| IBIS file stm32l4p5_wlcsp100_p.ibs
[IBIS ver]   4.2
[File name]  stm32l4p5_wlcsp100_p.ibs
[File Rev]   1.0
[Date]   04-10-2019
[Source]   Data Created at STMicroelectronics
[Notes]   File originated from ELDO simulations.
[Disclaimer] This information is for modeling purpose only and is
   not guaranted.
   The information is subject to change without notice.
[Copyright]  Copyright 2019 STMicroelectronics Inc.
|   Component stm32l4p5_wlcsp100_p
[Component] stm32l4p5_wlcsp100_p
[Manufacturer] STMicroelectronics
[Package]
| variable   typ   min   max
R_pkg  0  NA  NA
L_pkg  0  NA  NA
C_pkg  0  NA  NA
[Pin]   signal_name   model_name R_pin L_pin C_pin
A1 VDDUSB POWER
A10 VDD POWER
A2 PA15 io8prog2m25m50m120m_sudq_ft
A3 PD1 io8prog2m25m50m120m_sudq_ft
A4 VDD POWER
A5 PG10 io8prog2m25m50m120m_sudq_ft
A6 VDDIO2 POWER
A7 PB6 io8prog2m25m50m120m_sudq_i2c_ft
A8 PB9 io8prog2m25m50m120m_sudq_i2c_ft
A9 VDD12 POWER
B1 VSS GND
B10 PE3 io8prog2m25m50m120m_sudq_ft
B2 PA14 io8prog2m25m50m120m_sudq_ft
B3 PD0 io8prog2m25m50m120m_sudq_ft
B4 PD5 io8prog2m25m50m120m_sudq_ft
B5 PD6 io8prog2m25m50m120m_sudq_ft
B6 PG12 io8prog2m25m50m120m_sudq_ft
B7 PB7 io8prog2m25m50m120m_sudq_i2c_ft
B8 PB8 io8prog2m25m50m120m_sudq_i2c_ft
B9 VSS GND
C1 PA12 io8usblsfs_otg2
C10 VBAT POWER
C2 PA13 io8prog2m25m50m120m_sudq_ft
C3 PC10 io8prog2m25m50m120m_sudq_ft
C4 PC12 io8prog2m25m50m120m_sudq_ft
C5 PD4 io8prog2m25m50m120m_sudq_ft
C6 PD7 io8prog2m25m50m120m_sudq_ft
C7 PB5 io8prog2m25m50m120m_sudq_ft
C8 PE2 io8prog2m25m50m120m_sudq_ft
C9 PC13 io8prog2m25m50m120m_sudq_ft
D1 PA11 io8usblsfs_otg2
D10 PC14-OSC32_IN io8prog2m25m50m120m_sudq_ft
D2 PA10 io8usb_id_otg20_lcd4_ft_ms
D3 PA9 POWER
D4 PC11 io8prog2m25m50m120m_sudq_ft
D5 PD2 io8prog2m25m50m120m_sudq_ft
D6 PG9 io8prog2m25m50m120m_sudq_ft
D7 PH3-BOOT0 io8prog2m25m50m120m_sudq_ft
D8 PE6 io8prog2m25m50m120m_sudq_ft
D9 PC15-OSC32_OUT io8prog2m25m50m120m_sudq_ft
E1 PC8 io8prog2m25m50m120m_sudq_ft
E10 VSS GND
E2 PC9 io8prog2m25m50m120m_sudq_ft
E3 PA8 io8prog2m25m50m120m_sudq_ft
E4 PC7 io8prog2m25m50m120m_sudq_ft
E5 PG11 io8prog2m25m50m120m_sudq_ft
E6 PB4 io8prog2m25m50m120m_sudq_ft
E7 PE4 io8prog2m25m50m120m_sudq_ft
E8 PE5 io8prog2m25m50m120m_sudq_ft
E9 VDD POWER
F1 VDD POWER
F10 PH0-OSC_IN io8prog2m25m50m120m_sudq_ft
F2 PD15 io8prog2m25m50m120m_sudq_ft
F3 PD14 io8prog2m25m50m120m_sudq_ft
F4 PC6 io8prog2m25m50m120m_sudq_ft
F5 PB3 io8prog2m25m50m120m_sudq_ft
F6 PC3 io8prog2m25m50m120m_sudq_ft
F7 PC1 io8prog2m25m50m120m_sudq_i2c_ft
F8 NRST ioreset_ft_v33
F9 PH1-OSC_OUT io8prog2m25m50m120m_sudq_ft
G1 PD10 io8prog2m25m50m120m_sudq_ft
G10 PC0 io8prog2m25m50m120m_sudq_i2c_ft
G2 PD9 io8prog2m25m50m120m_sudq_ft
G3 PD8 io8prog2m25m50m120m_sudq_ft
G4 PE14 io8prog2m25m50m120m_sudq_ft
G5 PE13 io8prog2m25m50m120m_sudq_ft
G6 PA7 io8prog2m25m50m120m_sudq_ft
G7 PA1 io8prog2m25m50m120m_sudq_ft
G8 PA0 io8prog2m25m50m120m_sudq_ft
G9 PC2 io8prog2m25m50m120m_sudq_ft
H1 PB14 io8prog2m25m50m120m_sudq_i2c_ft
H10 VREF+ POWER
H2 PB13 io8prog2m25m50m120m_sudq_i2c_ft
H3 PB15 io8prog2m25m50m120m_sudq_ft
H4 PE15 io8prog2m25m50m120m_sudq_ft
H5 PE10 io8prog2m25m50m120m_sudq_ft
H6 PB0 io8prog2m25m50m120m_sudq_ft
H7 PA4 io8prog2m25m50m120m_sudq_ft
H8 PA2 io8prog2m25m50m120m_sudq_ft
H9 VSSA GND
J1 PB12 io8w_swp_lcd4_ft
J10 VDDA POWER
J2 VDD POWER
J3 PB11 io8prog2m25m50m120m_sudq_i2c_ft
J4 PE12 io8prog2m25m50m120m_sudq_ft
J5 PE9 io8prog2m25m50m120m_sudq_ft
J6 PB2 io8prog2m25m50m120m_sudq_ft
J7 PA5 io8prog2m25m50m120m_sudq_ft
J8 VDD POWER
J9 PA3 io8prog2m25m50m120m_sudq_ft
K1 VDD12 GND
K10 VSS GND
K2 VSS GND
K3 PB10 io8prog2m25m50m120m_sudq_i2c_ft
K4 PE11 io8prog2m25m50m120m_sudq_ft
K5 PE8 io8prog2m25m50m120m_sudq_ft
K6 PE7 io8prog2m25m50m120m_sudq_ft
K7 PB1 io8prog2m25m50m120m_sudq_ft
K8 PC4 io8prog2m25m50m120m_sudq_ft
K9 PA6 io8prog2m25m50m120m_sudq_ft
[Model Selector] io8prog2m25m50m120m_sudq_ft
iols8p_sudq_ft_pd_lv  "IO low speed, PD=40kOhm - 1P8V"
iols8p_sudq_ft_pu_lv  "IO low speed, PU=40kOhm - 1P8V"
iols8p_sudq_ft_lv  "IO low speed - 1P8V"
iols8p_sudq_ft_pd  "IO low speed, PD=40kOhm - 3P3V"
iols8p_sudq_ft_pu  "IO low speed, PU=40kOhm - 3P3V"
iols8p_sudq_ft  "IO low speed - 3P3V"
iofs8p_sudq_ft_pd_lv  "IO full speed, PD=40kOhm - 1P8V"
iofs8p_sudq_ft_pu_lv  "IO full speed, PU=40kOhm - 1P8V"
iofs8p_sudq_ft_lv  "IO full speed - 1P8V"
iofs8p_sudq_ft_pd  "IO full speed, PD=40kOhm - 3P3V"
iofs8p_sudq_ft_pu  "IO full speed, PU=40kOhm - 3P3V"
iofs8p_sudq_ft  "IO full speed - 3P3V"
ioms8p_sudq_ft_pd_lv  "IO medium speed, PD=40kOhm - 1P8V"
ioms8p_sudq_ft_pu_lv  "IO medium speed, PU=40kOhm - 1P8V"
ioms8p_sudq_ft_lv  "IO medium speed - 1P8V"
ioms8p_sudq_ft_pd  "IO medium speed, PD=40kOhm - 3P3V"
ioms8p_sudq_ft_pu  "IO medium speed, PU=40kOhm - 3P3V"
ioms8p_sudq_ft  "IO medium speed - 3P3V"
iohs8p_sudq_ft_pd_lv  "IO high speed, PD=40kOhm - 1P8V"
iohs8p_sudq_ft_pu_lv  "IO high speed, PU=40kOhm - 1P8V"
iohs8p_sudq_ft_lv  "IO high speed - 1P8V"
iohs8p_sudq_ft_pd  "IO high speed, PD=40kOhm - 3P3V"
iohs8p_sudq_ft_pu  "IO high speed, PU=40kOhm - 3P3V"
iohs8p_sudq_ft  "IO high speed - 3P3V"
[Model Selector] io8prog2m25m50m120m_sudq_i2c_ft
io8prog_1v8_i2c_pd  "5V Tol GPIO 1.8V range i2c functionality with pull down"
io8prog_1v8_i2c_pu  "5V Tol GPIO 1.8V range i2c functionality with pull up"
io8prog_1v8_i2c  "5V Tol GPIO 1.8V range i2c functionality"
io8prog_3v3_i2c_pd  "5V Tol GPIO 3.3V range i2c functionality with pull down"
io8prog_3v3_i2c_pu  "5V Tol GPIO 3.3V range i2c functionality with pull up"
io8prog_3v3_i2c  "5V Tol GPIO 3.3V range i2c functionality"
iols8p_sudq_ft_pd_lv  "IO low speed, PD=40kOhm - 1P8V"
iols8p_sudq_ft_pu_lv  "IO low speed, PU=40kOhm - 1P8V"
iols8p_sudq_ft_lv  "IO low speed - 1P8V"
iols8p_sudq_ft_pd  "IO low speed, PD=40kOhm - 3P3V"
iols8p_sudq_ft_pu  "IO low speed, PU=40kOhm - 3P3V"
iols8p_sudq_ft  "IO low speed - 3P3V"
iofs8p_sudq_ft_pd_lv  "IO full speed, PD=40kOhm - 1P8V"
iofs8p_sudq_ft_pu_lv  "IO full speed, PU=40kOhm - 1P8V"
iofs8p_sudq_ft_lv  "IO full speed - 1P8V"
iofs8p_sudq_ft_pd  "IO full speed, PD=40kOhm - 3P3V"
iofs8p_sudq_ft_pu  "IO full speed, PU=40kOhm - 3P3V"
iofs8p_sudq_ft  "IO full speed - 3P3V"
ioms8p_sudq_ft_pd_lv  "IO medium speed, PD=40kOhm - 1P8V"
ioms8p_sudq_ft_pu_lv  "IO medium speed, PU=40kOhm - 1P8V"
ioms8p_sudq_ft_lv  "IO medium speed - 1P8V"
ioms8p_sudq_ft_pd  "IO medium speed, PD=40kOhm - 3P3V"
ioms8p_sudq_ft_pu  "IO medium speed, PU=40kOhm - 3P3V"
ioms8p_sudq_ft  "IO medium speed - 3P3V"
iohs8p_sudq_ft_pd_lv  "IO high speed, PD=40kOhm - 1P8V"
iohs8p_sudq_ft_pu_lv  "IO high speed, PU=40kOhm - 1P8V"
iohs8p_sudq_ft_lv  "IO high speed - 1P8V"
iohs8p_sudq_ft_pd  "IO high speed, PD=40kOhm - 3P3V"
iohs8p_sudq_ft_pu  "IO high speed, PU=40kOhm - 3P3V"
iohs8p_sudq_ft  "IO high speed - 3P3V"
[Model Selector] io8w_swp_lcd4_ft
io8w_swp_classc  "Class C swp functionality"
io8w_swp_classb  "Class B swp functionality"
io8lsw_1v8_pd  "GPIO 1.8V range with pd io low speed"
io8lsw_1v8_pu  "GPIO 1.8V range with pu io low speed"
io8lsw_1v8  "GPIO 1.8V range io low speed"
io8lsw_3v3_pd  "GPIO 3.3V range with pd io low speed"
io8lsw_3v3_pu  "GPIO 3.3V range with pu io low speed"
io8lsw_3v3  "GPIO 3.3V range io low speed"
io8fsw_1v8_pd  "GPIO 1.8V range with pd io full speed"
io8fsw_1v8_pu  "GPIO 1.8V range with pu io full speed"
io8fsw_1v8  "GPIO 1.8V range io full speed"
io8fsw_3v3_pd  "GPIO 3.3V range with pd io full speed"
io8fsw_3v3_pu  "GPIO 3.3V range with pu io full speed"
io8fsw_3v3  "GPIO 3.3V range io full speed"
io8msw_1v8_pd  "GPIO 1.8V range with pd io medium speed"
io8msw_1v8_pu  "GPIO 1.8V range with pu io medium speed"
io8msw_1v8  "GPIO 1.8V range io medium speed"
io8msw_3v3_pd  "GPIO 3.3V range with pd io medium speed"
io8msw_3v3_pu  "GPIO 3.3V range with pu io medium speed"
io8msw_3v3  "GPIO 3.3V range io medium speed"
io8hsw_1v8_pd  "GPIO 1.8V range with pd io high speed"
io8hsw_1v8_pu  "GPIO 1.8V range with pu io high speed"
io8hsw_1v8  "GPIO 1.8V range io high speed"
io8hsw_3v3_pd  "GPIO 3.3V range with pd io high speed"
io8hsw_3v3_pu  "GPIO 3.3V range with pu io high speed"
io8hsw_3v3  "GPIO 3.3V range io high speed"
[Model Selector] io8usblsfs_otg2
usb_ls_pd  "USB Low Speed mode - Pull Down"
usb_ls_pu2  "USB Low Speed mode - Pull up 2"
usb_ls_pu  "USB Low Speed mode - Pull up"
usb_fs  "USB Low Speed mode"
usb_fs_pd  "USB Full Speed mode - Pull Down"
usb_fs_pu2  "USB Full Speed mode - Pull up 2"
usb_fs_pu  "USB Full Speed mode - Pull up"
[Model Selector] io8usb_id_otg20_lcd4_ft_ms
io8usbid_1v8_id_pu  "ID 1V8 range with pull up"
io8usbid_3v3_id_pu  "ID 3V3 range with pull up"
io8usbid_1v8_id  "ID 1V8 range"
io8usbid_3v3_id  "ID 3V3 range"
io8lsusbid_1v8_pd  "GPIO 1.8V range with pd io low speed"
io8lsusbid_1v8_pu  "GPIO 1.8V range with pu io low speed"
io8lsusbid_1v8  "GPIO 1.8V range io low speed"
io8lsusbid_3v3_pd  "GPIO 3.3V range with pd io low speed"
io8lsusbid_3v3_pu  "GPIO 3.3V range with pu io low speed"
io8lsusbid_3v3  "GPIO 3.3V range io low speed"
io8fsusbid_1v8_pd  "GPIO 1.8V range with pd io full speed"
io8fsusbid_1v8_pu  "GPIO 1.8V range with pu io full speed"
io8fsusbid_1v8  "GPIO 1.8V range io full speed"
io8fsusbid_3v3_pd  "GPIO 3.3V range with pd io full speed"
io8fsusbid_3v3_pu  "GPIO 3.3V range with pu io full speed"
io8fsusbid_3v3  "GPIO 3.3V range io full speed"
io8msusbid_1v8_pd  "GPIO 1.8V range with pd io medium speed"
io8msusbid_1v8_pu  "GPIO 1.8V range with pu io medium speed"
io8msusbid_1v8  "GPIO 1.8V range io medium speed"
io8msusbid_3v3_pd  "GPIO 3.3V range with pd io medium speed"
io8msusbid_3v3_pu  "GPIO 3.3V range with pu io medium speed"
io8msusbid_3v3  "GPIO 3.3V range io medium speed"
io8hsusbid_1v8_pd  "GPIO 1.8V range with pd io high speed"
io8hsusbid_1v8_pu  "GPIO 1.8V range with pu io high speed"
io8hsusbid_1v8  "GPIO 1.8V range io high speed"
io8hsusbid_3v3_pd  "GPIO 3.3V range with pd io high speed"
io8hsusbid_3v3_pu  "GPIO 3.3V range with pu io high speed"
io8hsusbid_3v3  "GPIO 3.3V range io high speed"
[Model Selector] ioreset_ft_v33
ioreset_1v2_pu  "RESET 1.2V range with PU"
ioreset_1v2  "RESET 1.2V range"
ioreset_1v8_pu  "RESET 1.8V range with PU"
ioreset_1v8  "RESET 1.8V range"
ioreset_3v3_pu  "RESET 3.3V range with PU"
ioreset_3v3  "RESET 3.3V range"
| Models and submodels in the file (97): iols8p_sudq_ft_pd_lv (I/O), iols8p_sudq_ft_pu_lv (I/O), iols8p_sudq_ft_lv (I/O), iols8p_sudq_ft_pd (I/O), iols8p_sudq_ft_pu (I/O), iols8p_sudq_ft (I/O), iofs8p_sudq_ft_pd_lv (I/O), iofs8p_sudq_ft_pu_lv (I/O), iofs8p_sudq_ft_lv (I/O), iofs8p_sudq_ft_pd (I/O), iofs8p_sudq_ft_pu (I/O), iofs8p_sudq_ft (I/O), ioms8p_sudq_ft_pd_lv (I/O), ioms8p_sudq_ft_pu_lv (I/O), ioms8p_sudq_ft_lv (I/O), ioms8p_sudq_ft_pd (I/O), ioms8p_sudq_ft_pu (I/O), ioms8p_sudq_ft (I/O), iohs8p_sudq_ft_pd_lv (I/O), iohs8p_sudq_ft_pu_lv (I/O), iohs8p_sudq_ft_lv (I/O), iohs8p_sudq_ft_pd (I/O), iohs8p_sudq_ft_pu (I/O), iohs8p_sudq_ft (I/O), io8prog_1v8_i2c_pd (I/O_open_drain), io8prog_1v8_i2c_pu (I/O_open_drain), io8prog_1v8_i2c (I/O_open_drain), io8prog_3v3_i2c_pd (I/O_open_drain), io8prog_3v3_i2c_pu (I/O_open_drain), io8prog_3v3_i2c (I/O_open_drain), io8w_swp_classc (I/O), io8w_swp_classb (I/O), io8lsw_1v8_pd (I/O), io8lsw_1v8_pu (I/O), io8lsw_1v8 (I/O), io8lsw_3v3_pd (I/O), io8lsw_3v3_pu (I/O), io8lsw_3v3 (I/O), io8fsw_1v8_pd (I/O), io8fsw_1v8_pu (I/O), io8fsw_1v8 (I/O), io8fsw_3v3_pd (I/O), io8fsw_3v3_pu (I/O), io8fsw_3v3 (I/O), io8msw_1v8_pd (I/O), io8msw_1v8_pu (I/O), io8msw_1v8 (I/O), io8msw_3v3_pd (I/O), io8msw_3v3_pu (I/O), io8msw_3v3 (I/O), io8hsw_1v8_pd (I/O), io8hsw_1v8_pu (I/O), io8hsw_1v8 (I/O), io8hsw_3v3_pd (I/O), io8hsw_3v3_pu (I/O), io8hsw_3v3 (I/O), usb_ls_pd (I/O), usb_ls_pu2 (I/O), usb_ls_pu (I/O), usb_fs (I/O), usb_fs_pd (I/O), usb_fs_pu2 (I/O), usb_fs_pu (I/O), io8usbid_1v8_id_pu (Input), io8usbid_3v3_id_pu (Input), io8usbid_1v8_id (Input), io8usbid_3v3_id (Input), io8lsusbid_1v8_pd (I/O), io8lsusbid_1v8_pu (I/O), io8lsusbid_1v8 (I/O), io8lsusbid_3v3_pd (I/O), io8lsusbid_3v3_pu (I/O), io8lsusbid_3v3 (I/O), io8fsusbid_1v8_pd (I/O), io8fsusbid_1v8_pu (I/O), io8fsusbid_1v8 (I/O), io8fsusbid_3v3_pd (I/O), io8fsusbid_3v3_pu (I/O), io8fsusbid_3v3 (I/O), io8msusbid_1v8_pd (I/O)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
